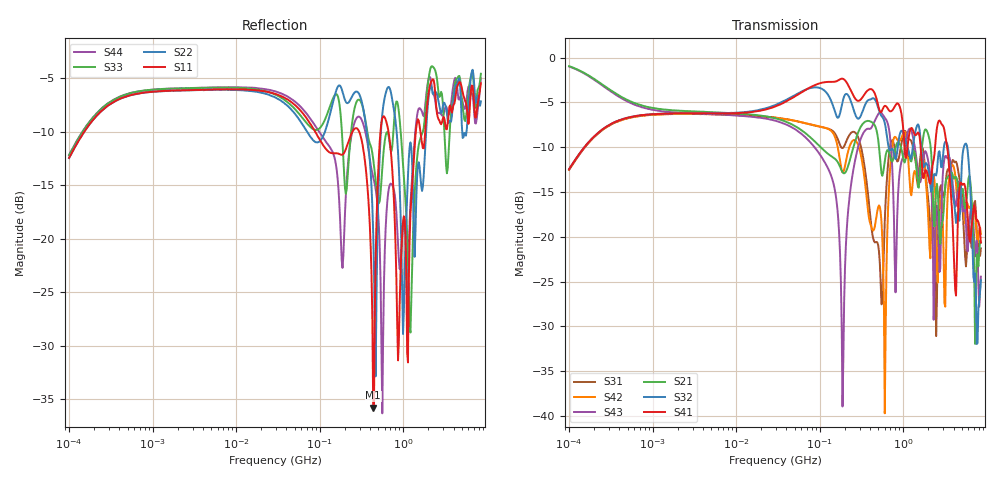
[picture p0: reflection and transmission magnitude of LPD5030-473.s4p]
# MHz S MA R 50
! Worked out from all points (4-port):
!   498 points, 100 kHz to 8.5 GHz, reference 50 ohm
!   strongest paths, dB at 100 kHz, 1.698 MHz, 29.49 MHz, 500.7 MHz, 8.5 GHz:
!     S41: -12.4, -6.2, -5.4, -5.3, -20.7
!     S32: -12.5, -6.2, -5.3, -5.6, -24.9
!     S21: -1.0, -5.9, -6.8, -9.1, -20.6
!     S43: -1.0, -6.1, -7.0, -6.3, -24.5
!     S42: -12.5, -6.3, -6.7, -16.7, -19.7
!     S31: -12.5, -6.3, -6.7, -20.9, -21.3
!   lowest |S11| = -35.8 dB at 436.5 MHz (marker M1), VSWR 1.03, Z = 49.3 - j1.43 ohm
!   |S11| at or under -10 dB: 297.1 MHz to 534.1 MHz (237 MHz wide, 57 % of centre); 665.9 MHz to 1.415 GHz (749.2 MHz wide, 72 % of centre); 1.605 GHz to 1.831 GHz (226.4 MHz wide, 13.2 % of centre)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
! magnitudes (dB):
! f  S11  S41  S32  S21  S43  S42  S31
! 100 kHz  -12.4  -12.4  -12.5  -1.0  -1.0  -12.5  -12.5
! 187.5 MHz  -12.1  -2.3  -4.9  -12.8  -38.9  -12.8  -10.1
! 436.5 MHz  -35.8  -3.7  -4.5  -7.3  -7.4  -19.3  -20.2
! 574.2 MHz  -8.6  -5.6  -6.8  -12.9  -6.4  -23.0  -24.2
! 866.1 MHz  -31.4  -5.1  -9.7  -9.4  -15.3  -9.3  -11.5
! 1.22 GHz  -17.7  -8.0  -11.3  -11.5  -8.0  -15.0  -9.2
! 8.5 GHz  -5.5  -20.7  -24.9  -20.6  -24.5  -19.7  -21.3
